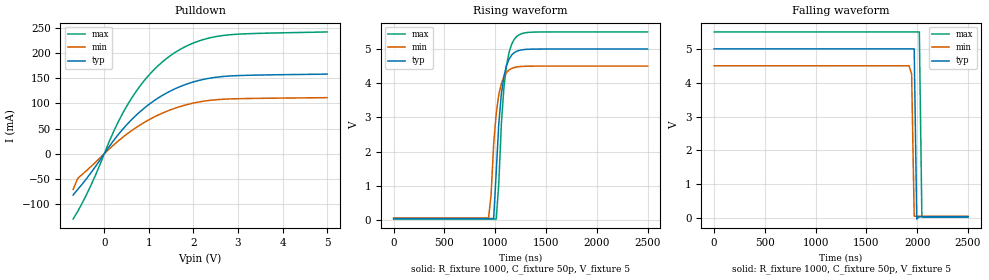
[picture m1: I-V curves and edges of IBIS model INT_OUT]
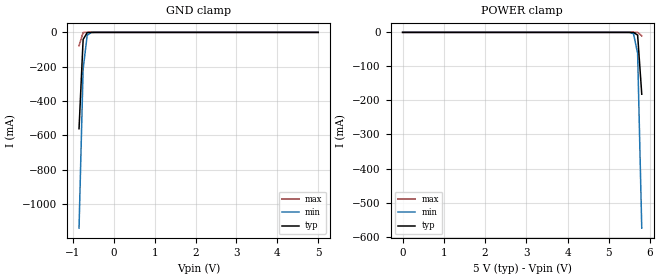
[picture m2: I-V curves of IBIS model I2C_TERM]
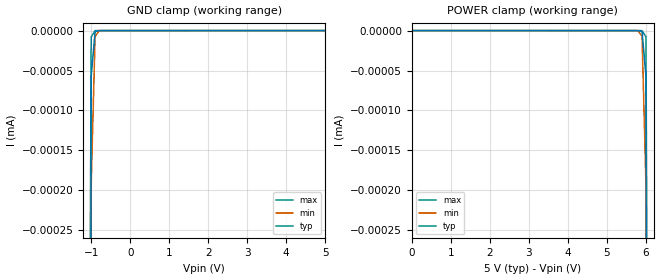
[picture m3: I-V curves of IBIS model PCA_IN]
|   NXP Semiconductors Inc.
|   Specialty Logic Products Group
|   IBIS model of PCA9543C
|   2-Channel I2C switch with
|   interrupt logic and reset
[IBIS Ver]   3.2
[Comment Char]   |_char
|  VDD: Typ: 5v, Min: 4.5v, 5.5v
[File name]   pca9543c_5v.ibs
[File Rev]   1.0
[Date]   Dec 12, 2007 11:55:50 AM
[Source]
Generated by Seshadri Venkataramanan with IbisToolKit at Tempe, AZ
[Notes]
[Disclaimer]
(C) Copyright 2007 NXP Semiconductors
All rights reserved
NXP Semiconductors (NXP) does not warrant that this model and any other
accompanying information (Model) accurately or fully represents the
operating characteristics and specifications of the semiconductor
products to which the Model relates.  Moreover, the Model is furnished
on an "as is" and with "all faults" basis, and without support or
warranty of any kind.  NXP disclaims all warranties, whether expressed
or implied or statutory, including without limitation all implied
warranties of non-infringement, merchantability and fitness for any
purpose, and those arising from a course of dealing or usage of trade.
NXP does not convey any license under its or any third party's patents,
copyrights or other intellectual property or proprietary rights.
You and your company assume any and all risks and liability arising out
of the application or use of the Model.
In no event shall NXP be liable for any direct, indirect, special,
consequential or incidental damages, however caused, whether in
warranty, contract or tort (including negligence), strict liability or
other legal theory, including, without limitation, for lost profits,
business interruption, or corruption or loss of data or information,
arising out of or in connection with the use of or the inability to use
the Model, even if NXP has been advised of the possibility of such
damages.
NXP provides the Model as a courtesy to our customers. You and your
company shall not distribute, convey, sell, or give the Model to anyone
else without receiving prior written permission from NXP.
NXP reserves the right to make changes without notice to the Model to
improve reliability, function, or design.
Please be aware that your receipt and subsequent use of the Model shall
serve as acceptance of these terms and conditions.  If you do not
accept these terms, return or destroy the Model immediately.
[Copyright]
2007
[Component]   PCA9543AD
Si_location Pin
Timing_location Pin
[Manufacturer]   NXP Semiconductors
[Package]
|   variable   typ   min   max
R_pkg   4.54E-02   4.38E-02   5.01E-02
L_pkg   2.31E-09   1.63E-09   3.26E-09
C_pkg   0.565E-12   0.437E-12   0.736E-12
|   SO14
[Pin] signal_name   model_name   R_pin   L_pin   C_pin
1   A0   PCA_IN   4.18E-02  3.26E-09  0.675E-12
2   A1   PCA_IN   5.01E-02  2.30E-09  0.574E-12
3   RESETB   PCA_IN   4.52E-02  1.71E-09  0.467E-12
4   INT0B   INT_IN   4.38E-02  1.63E-09  0.437E-12
5   SD0   I2C_TERM   4.52E-02  1.71E-09  0.465E-12
6   SC0   I2C_TERM   5.01E-02  2.30E-09  0.573E-12
7   VSS   GND   4.18E-02  3.26E-09  0.736E-12
8   INT1B   INT_IN   4.18E-02  3.26E-09  0.736E-12
9   SD1   I2C_TERM   5.01E-02  2.30E-09  0.573E-12
10   SC1   I2C_TERM   4.52E-02  1.71E-09  0.465E-12
11   INTB   INT_OUT   4.38E-02  1.63E-09  0.437E-12
12   SCL   I2C_TERM   4.52E-02  1.71E-09  0.467E-12
13   SDA   I2C_TERM   5.01E-02  2.30E-09  0.574E-12
14   VDD   POWER   4.18E-02  3.26E-09  0.736E-12
[Component]   PCA9543APW
Si_location Pin
Timing_location Pin
[Manufacturer]   NXP Semiconductors
[Package]
|   variable   typ   min   max
R_pkg   3.44E-02   2.80E-02   4.33E-02
L_pkg   1.83E-09   1.36E-09   2.32E-09
C_pkg   0.380E-12   0.302E-12   0.442E-12
|   TSSOP14
[Pin] signal_name   model_name   R_pin   L_pin   C_pin
1   A0   PCA_IN   3.46E-02  2.32E-09  0.423E-12
2   A1   PCA_IN   4.33E-02  2.04E-09  0.441E-12
3   RESETB   PCA_IN   2.80E-02  1.36E-09  0.307E-12
4   INT0B   INT_IN   2.88E-02  1.38E-09  0.302E-12
5   SD0   I2C_TERM   2.80E-02  1.36E-09  0.308E-12
6   SC0   I2C_TERM   4.33E-02  2.04E-09  0.441E-12
7   VSS   GND   3.46E-02  2.32E-09  0.433E-12
8   INT1B   INT_IN   3.46E-02  2.32E-09  0.433E-12
9   SD1   I2C_TERM   4.33E-02  2.04E-09  0.441E-12
10   SC1   I2C_TERM   2.80E-02  1.36E-09  0.308E-12
11   INTB   INT_OUT   2.88E-02  1.38E-09  0.302E-12
12   SCL   I2C_TERM   2.80E-02  1.36E-09  0.308E-12
13   SDA   I2C_TERM   4.33E-02  2.04E-09  0.442E-12
14   VDD   POWER   3.46E-02  2.31E-09  0.433E-12
[Series Pin Mapping] pin_2 model_name   function_table_group
5   13   PCA_SW   1
6   12   PCA_SW   1
9   13   PCA_SW   2
10   12   PCA_SW   2
[Series Switch Groups]
|   Default both off
Off 1 2 /
|   Other possibilities
On 1 /
On 2 /
[Model]   PCA_SW
Model_type Series_switch
C_comp   0.5p   0.5p   0.5p
[Temperature Range] 27   -40   85
[Voltage Range]   3.3   2.3   5.5
[Pullup Reference]  3.3   2.3   5.5
[Pulldown Reference]0   0   0
[On]
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[Off]
|   variable   R(typ)   R(min)   R(max)
[R Series]   1e06   1e06   1e06
|[End   PCA_SW
| Models and submodels in the file (5): INT_OUT (Open_drain), I2C_TERM (Terminator), PCA_IN (Input), INT_IN (Input), PCA_SW (Series_switch)
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[Model]   INT_OUT
Model_type Open_drain
Vref=5
Vmeas=2.5
Rref=1000
Cref=1p
C_comp   2.2p   2p   2.3p
[Model Spec]
Vmeas   2.5   2.25   2.75
[Temperature Range] 27   85   -40
[Voltage Range]   5   4.5   5.5
[Pullup Reference]  5   4.5   5.5
[Pulldown Reference]0   0   0
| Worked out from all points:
|   slope of the pulldown table from 0 to 0.75 V, typ, clamps not added: 9.45 ohm
|   falling waveform, R_fixture 1000, C_fixture 50p, V_fixture 5: 20-80 % time 14.9ns typ, 16ns min, 15.2ns max; typ from 5 V to 0.038 V
|   rising waveform, R_fixture 1000, C_fixture 50p, V_fixture 5: 20-80 % time 73.4ns typ, 70ns min, 70.7ns max; typ from 0.038 V to 5 V
[Pulldown]
-700mV    -82.56mA   -71.37mA   -130.3mA
-600mV    -71.48mA   -49.68mA   -115.5mA
-300mV    -38.11mA   -25.72mA   -63.02mA
200mV     25.14mA    16.62mA    42.35mA
500mV     57.27mA    38.53mA    94.25mA
700mV     75.3mA     51.18mA    122.3mA
1V        97.92mA    67.41mA    156.4mA
1.5V      125.5mA    87.77mA    196.3mA
2V        142.9mA    100.7mA    220.4mA
2.6V      153.1mA    108mA      234.6mA
3.2V      156mA      109.8mA    238.8mA
5V        158.4mA    111.5mA    242.5mA
[Falling Waveform]
R_fixture=1000
C_fixture=50p
V_fixture=5
V_fixture_min=4.5
V_fixture_max=5.5
0s        5V         4.5V       5.5V
1.919us   5V         4.5V       5.5V
1.944us   5V         4.253V     5.5V
1.97us    5V         52.05mV    5.5V
1.995us   -30mV      51.75mV    5.5V
2.02us    37.69mV    51.74mV    5.5V
2.045us   37.68mV    51.75mV    25.76mV
2.5us     37.68mV    51.74mV    24.26mV
[Rising Waveform]
R_fixture=1000
C_fixture=50p
V_fixture=5
V_fixture_min=4.5
V_fixture_max=5.5
0s        37.68mV    51.74mV    24.26mV
934.3ns   37.72mV    51.77mV    24.33mV
959.6ns   37.73mV    743.7mV    24.33mV
984.8ns   37.77mV    2.22V      24.34mV
1.01us    1.406V     3.117V     24.37mV
1.035us   2.821V     3.662V     1.068V
1.086us   4.2V       4.192V     3.873V
1.136us   4.706V     4.387V     4.903V
1.212us   4.935V     4.475V     5.368V
2.5us     5V         4.5V       5.5V
[Ramp]
R_load=1000
dV/dt_r   2.977E+0/1.199E-9   2.965E+0/1.175E-9   2.987E+0/1.163E-9
dV/dt_f   2.977E+0/1.097E-9   2.965E+0/1.187E-9   2.987E+0/7.196E-10
|[End   INT_OUT
| [End   I2C_TERM
|  [End   I2C_TERM
[Model]   I2C_TERM
Model_type Terminator
C_comp   9.5p   9.5p   9.5p
[Temperature Range] 27   85   -40
[Voltage Range]   5   4.5   5.5
[Pullup Reference]  5   4.5   5.5
[Pulldown Reference]0   0   0
[POWER Clamp Reference]5   4.5   5.5
[GND Clamp Reference]0   0   0
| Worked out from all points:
|   GND clamp passes 1 mA (typ) near -0.62 V on its own axis
[GND Clamp]
|   -6.000000E-1   -1.554225E-1   -1.242642E-1   -2.666059E-1
|   -5.000000E-1   -1.602113E-1   -1.179351E-1   -2.662641E-1
|   -4.000000E-1   -1.574088E-1   -1.099432E-1   -2.800035E-1
-850mV    -561.7mA   -1.141A    -77.71mA
-750mV    -41.44mA   -214.7mA   -986.6uA
-650mV    -1.335mA   -16.09mA   -6.931uA
-550mV    -28.83uA   -825.5uA   -47.83nA
-450mV    -604nA     -33.09uA   -373.8pA
5V        449pA      492.4pA    471.4pA
[POWER Clamp]
0V        449pA      492.4pA    471.4pA
5.4V      -87.32nA   -6.549uA   -66.94pA
5.5V      -4.169uA   -166.5uA   -4.015nA
5.6V      -198.2uA   -3.861mA   -575.5nA
5.7V      -8.107mA   -61.58mA   -83.36uA
5.8V      -181.7mA   -575.2mA   -10.26mA
[Model]   PCA_IN
Model_type Input
Vinh=2.1
Vinl=0.9
C_comp   1.73p   1.73p   1.73p
[Temperature Range] 27   85   -40
[Voltage Range]   5   4.5   5.5
[POWER Clamp Reference]5   4.5   5.5
[GND Clamp Reference]0   0   0
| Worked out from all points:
|   GND clamp passes 1 mA (typ) near -1.21 V on its own axis
[GND Clamp]
-2V       -10.17A    -9.093A    -11.52A
-1.1V     -2.721uA   -4.917uA   -1.144uA
-1V       -56.96nA   -192.5nA   -7.885nA
-900mV    -1.193nA   -7.54nA    -55.23pA
-800mV    -25.76pA   -296pA     -1.175pA
-700mV    -1.223pA   -12.26pA   -702.6fA
5V        5pA        5pA        5pA
[POWER Clamp]
0V        5pA        5pA        5pA
5.7V      -1.223pA   -12.26pA   -702.6fA
5.8V      -25.76pA   -296pA     -1.175pA
5.9V      -1.193nA   -7.54nA    -55.23pA
6V        -56.96nA   -192.5nA   -7.885nA
6.1V      -2.721uA   -4.917uA   -1.144uA
7V        -10.17A    -9.093A    -11.52A
